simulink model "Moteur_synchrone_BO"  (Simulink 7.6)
settings: Solver=ode15s  StartTime=0.0  StopTime=0.5  MaxStep=1/60  RelTol=1e-4  AbsTol=1e-4
InitFcn:
  | clear all
  | close all
  | delete *.mat
  | clc
StopFcn:
  | close all
  | load Istator_Vitesse.mat
  | plotyy(x(1,:),x(2,:), x(1,:),x(3,:))
  | title('Courant statorique et vitesse de rotation')
  | grid
  | xlabel('temps')
undefined symbols (not defined in the file or in its folder): by, established, Flux, linkage, magnets, V
libraries: powerlib x4, powerlib_extras x1

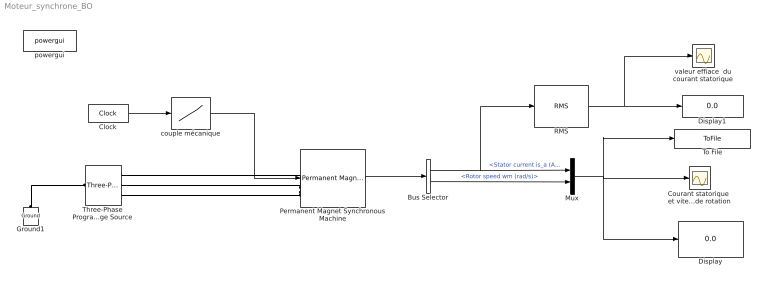
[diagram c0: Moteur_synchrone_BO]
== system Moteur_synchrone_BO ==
  Bus Selector : BusSelector  OutputSignals=Stator current is_a (A),Rotor speed wm (rad/s)
  Clock : Clock
  Courant statorique  et vitesse de rotation : Scope
  Display : Display
  Display1 : Display
  Ground1 : powerlib/Elements/Ground  DialogController=POWERSYS.PowerSysDialog  PhysicalDomain=powersysdomain  SubClassName=unknown  LeftPortType=p1  RightPortType=p1  LConnTagsString=a
  Mux : Mux  Inputs=2
  Permanent Magnet Synchronous Machine : powerlib/Machines/Permanent Magnet Synchronous Machine  DialogController=POWERSYS.PowerSysDialog  SystemSampleTime=-1  FluxDistribution=Sinusoidal  MechanicalLoad=Torque Tm  PresetModel=No  ShowDetailedParameters=on  Resistance=2.8750  Inductance=8.5e-3  dqInductances=[8.5e-3,8.5e-3]  MachineConstant=Flux linkage established by magnets (V.s)  Flux=0.175  VoltageCst=126.966  TorqueCst=1.05  Flat=120  Mechanical=[0.0008 0.001 4]  PolePairs=4  InitialConditions=[0,0, 0,0]  TsPowergui=0  TsBlock=-1
  RMS : powerlib_extras/Measurements/RMS  DialogController=POWERSYS.PowerSysDialog  SystemSampleTime=-1  f1=60
  Three-Phase Programmable  Voltage Source : powerlib/Electrical Sources/Three-Phase Programmable Voltage Source  DialogController=POWERSYS.PowerSysDialog  SystemSampleTime=-1  PositiveSequence="[380  0 60]"  VariationEntity=Amplitude  VariationType=Step  VariationStep=0.5  VariationRate=10  VariationMagnitude=0.3  VariationFrequency=2  VariationTiming=[10 30]  VariationPhaseA=off  Amplitudes=[1 0.8 1.2 1.0]  TimeValues=[0 0.1 0.15 0.2]  HarmonicGeneration=off  HarmonicA=[3 0.2 -25 0]  HarmonicB=[2 0.15 35 2]  Timing="[0.05  3]"
  To File : ToFile  Filename=Istator_Vitesse  MatrixName=x
  couple mécanique : Lookup  InputValues=[0 0.2 0.201 0.5]  Table=[0 0 50 50]
  powergui : powerlib/powergui  Priority=2  SystemSampleTime=-1  SimulationMode=Discrete  SampleTime=1e-5  frequency=60  SPID=off  DisableSnubberDevices=off  DisableRonSwitches=off  DisableVfSwitches=off  SwTol=0  Interpol=off  frequencyindice=60  echomessages=off  HookPort=off  DisplayEquations=off  FunctionMessages=off  EnableUseOfTLC=off  x0status=blocks  RestoreLinks=warning  ResistiveCurrentMeasurement=off  Frange=[0:2:500]  Ylog=off  Xlog=on  ShowGrid=off  save=off  variable=ZData  ZoomFFT=on  StartTime=0.0  cycles=1  DisplayStyle=1  fundamental=60  FreqAxis=off  MaxFrequency=1000  frequencyindicesteady=1  RmsSteady=1  display=off  Ts=0  methode=off
  valeur effiace  du courant statorique : Scope
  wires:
  Permanent Magnet Synchronous Machine/1 -> Bus Selector/1
  Mux/1 -> Courant statorique  et vitesse de rotation/1, To File/1, Display/1
  Bus Selector/1 -> Mux/1, RMS/1  "<Stator current is_a (A)>"
  Bus Selector/2 -> Mux/2  "<Rotor speed wm (rad/s)>"
  couple mécanique/1 -> Permanent Magnet Synchronous Machine/1
  Clock/1 -> couple mécanique/1
  RMS/1 -> Display1/1, valeur effiace  du courant statorique/1
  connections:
  Permanent Magnet Synchronous Machine/LConn1 -- Three-Phase Programmable  Voltage Source/RConn1
  Permanent Magnet Synchronous Machine/LConn2 -- Three-Phase Programmable  Voltage Source/RConn2
  Permanent Magnet Synchronous Machine/LConn3 -- Three-Phase Programmable  Voltage Source/RConn3
  Ground1/LConn1 -- Three-Phase Programmable  Voltage Source/LConn1
